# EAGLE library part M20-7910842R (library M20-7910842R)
2.54mm (0.1") Pitch SIL Horizontal SMT Socket Assembly, selective gold + tin (Tape & Reel packing), 8 contacts Source: Datasheet
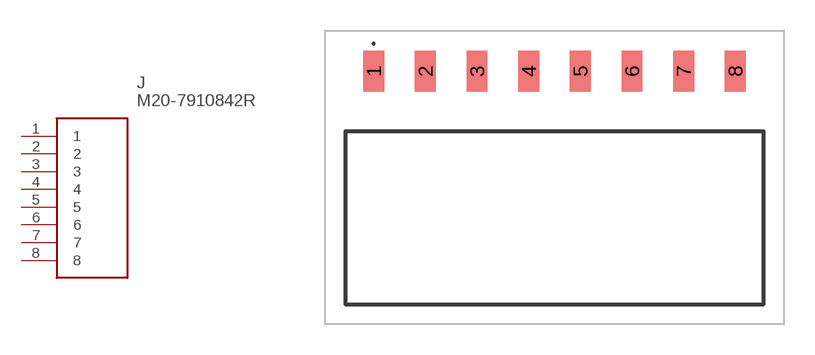
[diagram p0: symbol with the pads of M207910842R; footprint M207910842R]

Designator prefix J

## M20-7910842R (Description: 2.54mm (0.1") Pitch SIL Horizontal SMT Socket Assembly, selective gold + tin (Tape & Reel packing), 8 contacts; Height: 2.65mm; Manufacturer_Name: Harwin; Manufacturer_Part_Number: M20-7910842R; Mouser_Part_Number: 855-M20-7910842R; Mouser_Price-Stock: https://www.mouser.co.uk/ProductDetail/Harwin/M20-7910842R?qs=k41KVqW3ympJ6ZCQNkwKKw%3D%3D)  [M207910842R]
1  1
2  2
3  3
4  4
5  5
6  6
7  7
8  8

## Footprint M207910842R (pad centres in mm)
M20-7910842R-4
smd 1.02 x 2: 1 -8.89,7.224; 2 -6.35,7.224; 3 -3.81,7.224; 4 -1.27,7.224; 5 1.27,7.224; 6 3.81,7.224; 7 6.35,7.224; 8 8.89,7.224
